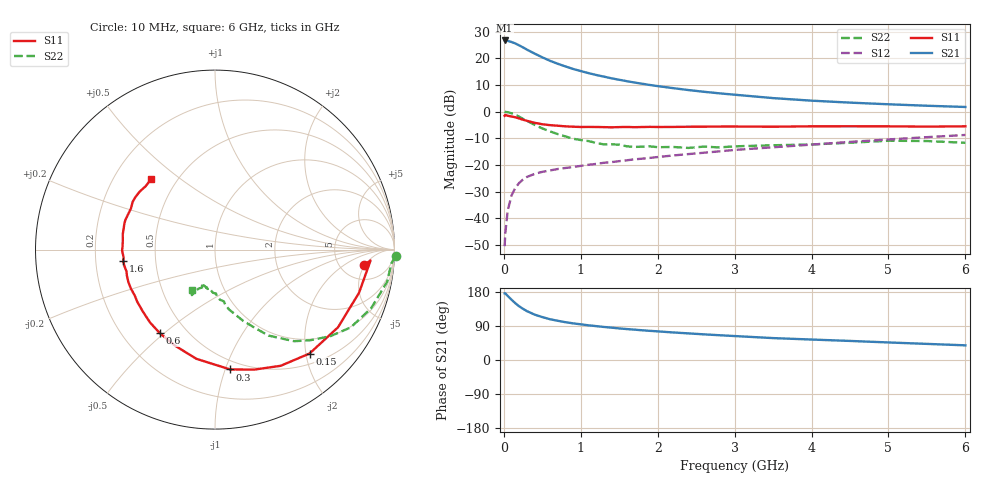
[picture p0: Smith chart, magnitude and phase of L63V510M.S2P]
!  INFINEON TECHNOLOGIES Small Signal Semiconductors
! BFR380L3 , Si-NPN RF-Transistor in TSLP-3-1
!  Vce=3.5 V,  Ic=10 mA
! Common Emitter S-Parameters:  07. March 2005
#  GHz  S  MA  R  50
! f  S11  S21  S12  S22
! GHz  Mag  Ang  Mag  Ang  Mag  Ang  Mag  Ang
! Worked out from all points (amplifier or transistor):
!   36 points, 10 MHz to 6 GHz, reference 50 ohm
!   highest |S21| = 26.7 dB at 10 MHz (marker M1)
!   |S21| within 3 dB of that: start of sweep to 273.8 MHz
!   unconditionally stable (mu >= 1): 2.285 GHz to 4.711 GHz
!   at 250 MHz: K = 0.24, MSG = 24.8 dB, |S12| = -25.4 dB
!   at 1.4 GHz: K = 0.87, MSG = 15.7 dB, |S12| = -18.9 dB
!   at 6 GHz: K = 0.96, MSG = 5.2 dB, |S12| = -8.7 dB
!   S11 on the Smith chart (normalised r, x): 10 MHz: 8.51, -4.79; 150 MHz: 0.69, -2.07; 300 MHz: 0.43, -1.04; 600 MHz: 0.36, -0.48; 1.6 GHz: 0.32, -0.06; 6 GHz: 0.36, +0.39
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0.01  0.8365 -5.8  21.6 175.9  0.003 82.8  1.007 -2.1
0.02  0.8687 -4.0  21.53 175.7  0.0054 93.0  0.9858 -4.4
0.05  0.8378 -16.7  21.19 169.1  0.0139 85.8  0.9757 -10.6
0.1  0.8106 -32.3  20.18 159.1  0.0268 73.9  0.9297 -20.5
0.15  0.7828 -47.7  18.96 149.7  0.0374 67.8  0.872 -29.8
0.2  0.7437 -60.5  17.44 141.6  0.0461 63.5  0.8044 -36.8
0.25  0.7034 -71.9  15.98 135.0  0.0534 57.8  0.7315 -43.7
0.3  0.673 -82.8  14.56 129.0  0.0596 55.0  0.6743 -49.2
0.4  0.6172 -99.7  12.25 119.8  0.0679 50.7  0.5643 -58.1
0.5  0.5798 -112.6  10.43 113.2  0.0742 48.4  0.4846 -63.4
0.6  0.5577 -123.6  8.977 107.6  0.0789 47.5  0.4264 -68.5
0.7  0.5439 -131.8  7.901 103.5  0.0839 47.2  0.3796 -72.6
0.8  0.5297 -139.4  7.041 99.8  0.0877 47.4  0.3427 -76.8
1.1  0.5164 -155.1  5.277 91.5  0.1008 49.5  0.2804 -84.4
1.4  0.5077 -166.2  4.211 85.4  0.1131 51.6  0.2442 -90.1
1.6  0.5156 -172.8  3.718 81.6  0.1224 53.0  0.2235 -96.6
2.2  0.5161 174.4  2.756 72.7  0.1506 56.5  0.2174 -102.2
2.8  0.5254 163.9  2.204 65.4  0.1799 59.0  0.2131 -109.9
3.5  0.5212 154.1  1.793 57.8  0.2144 59.4  0.234 -112.5
4.5  0.5313 146.8  1.475 50.3  0.2704 60.5  0.2608 -115.4
5.5  0.5235 137.7  1.289 42.5  0.332 58.7  0.2808 -117.5
6  0.53 132.1  1.222 38.7  0.3652 57.2  0.2599 -119.1
